|   TEXAS INSTRUMENTS INCORPORATED
|   Standard Linear and Logic
|   IBIS Model of SN74LVTH16244A
|   3.3-V ABT 16-BIT BUFFERS/DRIVERS
|   WITH 3-STATE OUTPUTS
|   TSSOP 48-pin package (DGG)
|   TVSOP 48-pin package (DGV)
|   SSOP 48-pin package (DL)
|   VFBGA 56-pin package (GQL)
[IBIS Ver]   3.2
[Comment char] |_char
[File Name]   sn74lvth16244a.ibs
[File Rev]   1.2 | a_die
[Date]   12/08/04
[Source]   File originated at Texas Instruments, Inc
[Notes]   The following is a sample IBIS file for the SN74LVTH16244A.
   - FILE REV HISTORY
   - 1.2 Re-Release IBIS file on 12/30/04
|   - All test data contained in this file are derived from
|   actual measurement.
|   - The measurement used DGG package.
|   - We have data across voltage and temperature, but not across
|   process.
|   - Since this is a BiCMOS process, we have irregular trend for the
|   curves at high and low temperatures. This data was taken with
|   high temperature for strong case and low for weak case.
|   - Due to presence of BUS-HOLD at input, GND-CLAMP curves
|   have non-monotonic warnings.
|   - Due to the fact that the Device is 5-V Input/Output
|   tolarent, the output model has some Non-Monotonic Warnings.
|   - Power clamp data deleted as there is no power-clamp diode.
|   - File created by Nobuhisa Ohtsubo, TIJ SLL Product Engineering.
|*   Property of Texas Instruments Incorporated.  Unauthorized   *
|*   reproduction and/or distribution is strictly prohibited.   *
|*   This product is protected under copyright law.   *
|*   Created 1998, (C) Copyright 1998, Texas Instruments Inc.,   *
|*   All Rights Reserved   *
|*   UNLESS THERE IS A SIGNED, WRITTEN AGREEMENT TO THE   *
|*   CONTRARY, TEXAS INSTRUMENTS ("TI") IS PROVIDING THE SPICE   *
|*   MODELS "AS IS" AND WITHOUT ANY WARRANTY, EXPRESSED OR   *
|*   IMPLIED.  TI assumes no liability for:   *
|*   1) the accuracy of the IBIS models provided to your   *
|*   company;   *
|*   2) the proper functioning of these IBIS models in your   *
|*   design or for any resulting applications; or   *
|*   3) infringement of patents, copyrights or intellectual   *
|*   property rights resulting from your use of these   *
|*   IBIS models.   *
|*   TI provides IBIS Models as a service to our customers.   *
|*   You and your company shall not distribute, sell or give   *
|*   these models to anyone else without prior written   *
|*   permission from TI.   *
|*   TI reserves the right to make changes to our products or   *
|*   to discontinue any semiconductor product or service   *
|*   without notice, and advises our customers to obtain the   *
|*   latest version of relevant information to verify, before   *
|*   placing orders, that the information being relied on is   *
|*   current.   *
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[Component]   LVTH16244A_DGG
[manufacturer]   Texas Instruments, Inc.
[Package]
|   typ   min   max
R_pkg   0.044   0.038   0.051
L_pkg   3.019nH   2.486nH   4.099nH
C_pkg   0.507pF   0.334pF   0.809pF
[Pin] signal_name  model_name   R_pin   L_pin   C_pin
1   1NOE   LVTH16244A_OE   0.041   4.017nH   0.759pF
2   1Y1   LVTH16244A_OUT   0.042   3.737nH   0.792pF
3   1Y2   LVTH16244A_OUT   0.042   3.48nH   0.661pF
4   GND   GND   0.038   3.131nH   0.575pF
5   1Y3   LVTH16244A_OUT   0.047   3.122nH   0.566pF
6   1Y4   LVTH16244A_OUT   0.043   2.948nH   0.504pF
7   VCC   POWER   0.045   2.845nH   0.397pF
8   2Y1   LVTH16244A_OUT   0.049   2.835nH   0.394pF
9   2Y2   LVTH16244A_OUT   0.048   2.715nH   0.378pF
10   GND   GND   0.050   2.664nH   0.363pF
11   2Y3   LVTH16244A_OUT   0.050   2.585nH   0.348pF
12   2Y4   LVTH16244A_OUT   0.049   2.55nH   0.337pF
13   3Y1   LVTH16244A_OUT   0.049   2.541nH   0.336pF
14   3Y2   LVTH16244A_OUT   0.050   2.574nH   0.348pF
15   GND   GND   0.049   2.618nH   0.359pF
16   3Y3   LVTH16244A_OUT   0.046   2.671nH   0.375pF
17   3Y4   LVTH16244A_OUT   0.045   2.754nH   0.389pF
18   VCC   POWER   0.044   2.823nH   0.450pF
19   4Y1   LVTH16244A_OUT   0.042   2.968nH   0.503pF
20   4Y2   LVTH16244A_OUT   0.051   3.108nH   0.535pF
21   GND   GND   0.042   3.175nH   0.587pF
22   4Y3   LVTH16244A_OUT   0.041   3.449nH   0.678pF
23   4Y4   LVTH16244A_OUT   0.044   3.766nH   0.804pF
24   4NOE   LVTH16244A_OE   0.043   4.065nH   0.761pF
25   3NOE   LVTH16244A_OE   0.041   3.994nH   0.757pF
26   4A4   LVTH16244A_IN   0.039   3.649nH   0.789pF
27   4A3   LVTH16244A_IN   0.038   3.362nH   0.660pF
28   GND   GND   0.038   3.082nH   0.574pF
29   4A2   LVTH16244A_IN   0.044   2.99nH   0.522pF
30   4A1   LVTH16244A_IN   0.041   2.917nH   0.495pF
31   VCC   POWER   0.043   2.82nH   0.448pF
32   3A4   LVTH16244A_IN   0.043   2.699nH   0.385pF
33   3A3   LVTH16244A_IN   0.045   2.628nH   0.372pF
34   GND   GND   0.046   2.556nH   0.356pF
35   3A2   LVTH16244A_IN   0.046   2.495nH   0.344pF
36   3A1   LVTH16244A_IN   0.047   2.487nH   0.334pF
37   2A4   LVTH16244A_IN   0.047   2.49nH   0.335pF
38   2A3   LVTH16244A_IN   0.046   2.486nH   0.343pF
39   GND   GND   0.045   2.566nH   0.356pF
40   2A2   LVTH16244A_IN   0.044   2.639nH   0.374pF
41   2A1   LVTH16244A_IN   0.043   2.701nH   0.386pF
42   VCC   POWER   0.043   2.817nH   0.450pF
43   1A4   LVTH16244A_IN   0.041   2.935nH   0.501pF
44   1A3   LVTH16244A_IN   0.047   3.035nH   0.529pF
45   GND   GND   0.043   3.171nH   0.589pF
46   1A2   LVTH16244A_IN   0.040   3.415nH   0.682pF
47   1A1   LVTH16244A_IN   0.043   3.741nH   0.809pF
48   2NOE   LVTH16244A_OE   0.044   4.099nH   0.764pF
|   TVSOP  48-pin (DGV) package
[Component]   LVTH16244A_DGV
[manufacturer]   Texas   Instruments, Inc.
[Package]
|   typ   min   max
R_pkg   0.063   0.043   0.09
L_pkg   3.077nH   2.377nH   4.305nH
C_pkg   0.387pF   0.281pF   0.565pF
[Pin] signal_name   model_name   R_pin   L_pin   C_pin
1   1NOE   LVTH16244A_OE   0.082   4.277nH   0.562pF
2   1Y1   LVTH16244A_OUT   0.090   4.02nH   0.554pF
3   1Y2   LVTH16244A_OUT   0.087   3.719nH   0.478pF
4   GND   GND   0.087   3.456nH   0.417pF
5   1Y3   LVTH16244A_OUT   0.076   3.207nH   0.411pF
6   1Y4   LVTH16244A_OUT   0.044   2.929nH   0.390pF
7   VCC   POWER   0.046   2.803nH   0.335pF
8   2Y1   LVTH16244A_OUT   0.047   2.683nH   0.321pF
9   2Y2   LVTH16244A_OUT   0.048   2.579nH   0.311pF
10   GND   GND   0.049   2.505nH   0.302pF
11   2Y3   LVTH16244A_OUT   0.048   2.4nH   0.289pF
12   2Y4   LVTH16244A_OUT   0.051   2.4nH   0.283pF
13   3Y1   LVTH16244A_OUT   0.051   2.4nH   0.283pF
14   3Y2   LVTH16244A_OUT   0.050   2.433nH   0.291pF
15   GND   GND   0.048   2.46nH   0.298pF
16   3Y3   LVTH16244A_OUT   0.048   2.585nH   0.312pF
17   3Y4   LVTH16244A_OUT   0.046   2.652nH   0.319pF
18   VCC   POWER   0.045   2.787nH   0.336pF
19   4Y1   LVTH16244A_OUT   0.046   2.962nH   0.394pF
20   4Y2   LVTH16244A_OUT   0.074   3.208nH   0.409pF
21   GND   GND   0.087   3.488nH   0.417pF
22   4Y3   LVTH16244A_OUT   0.087   3.741nH   0.478pF
23   4Y4   LVTH16244A_OUT   0.089   3.99nH   0.546pF
24   4NOE   LVTH16244A_OE   0.084   4.305nH   0.557pF
25   3NOE   LVTH16244A_OE   0.082   4.286nH   0.565pF
26   4A4   LVTH16244A_IN   0.086   3.933nH   0.554pF
27   4A3   LVTH16244A_IN   0.086   3.699nH   0.475pF
28   GND   GND   0.089   3.522nH   0.420pF
29   4A2   LVTH16244A_IN   0.079   3.234nH   0.413pF
30   4A1   LVTH16244A_IN   0.043   2.88nH   0.385pF
31   VCC   POWER   0.045   2.779nH   0.332pF
32   3A4   LVTH16244A_IN   0.045   2.636nH   0.317pF
33   3A3   LVTH16244A_IN   0.047   2.553nH   0.309pF
34   GND   GND   0.048   2.468nH   0.298pF
35   3A2   LVTH16244A_IN   0.050   2.424nH   0.290pF
36   3A1   LVTH16244A_IN   0.050   2.377nH   0.281pF
37   2A4   LVTH16244A_IN   0.050   2.387nH   0.281pF
38   2A3   LVTH16244A_IN   0.050   2.431nH   0.290pF
39   GND   GND   0.048   2.475nH   0.299pF
40   2A2   LVTH16244A_IN   0.048   2.557nH   0.309pF
41   2A1   LVTH16244A_IN   0.047   2.671nH   0.319pF
42   VCC   POWER   0.046   2.804nH   0.334pF
43   1A4   LVTH16244A_IN   0.044   2.935nH   0.390pF
44   1A3   LVTH16244A_IN   0.074   3.203nH   0.412pF
45   GND   GND   0.085   3.444nH   0.416pF
46   1A2   LVTH16244A_IN   0.085   3.723nH   0.477pF
47   1A1   LVTH16244A_IN   0.090   4.012nH   0.547pF
48   2NOE   LVTH16244A_OE   0.083   4.288nH   0.558pF
|   SSOP 48-pin (DL) package
[Component]   LVTH16244A_DL
[manufacturer]   Texas Instruments, Inc.
[Package]
|   typ   min   max
R_pkg   0.048   0.038   0.053
L_pkg   6.046nH   5.084nH   7.968nH
C_pkg   0.813pF   0.569pF   1.157pF
[Pin] signal_name   model_name   R_pin   L_pin   C_pin
1   1NOE   LVTH16244A_OE   0.046   7.968nH   1.017pF
2   1Y1   LVTH16244A_OUT   0.044   7.299nH   1.157pF
3   1Y2   LVTH16244A_OUT   0.043   6.765nH   1.058pF
4   GND   GND   0.041   6.269nH   0.933pF
5   1Y3   LVTH16244A_OUT   0.038   5.856nH   0.829pF
6   1Y4   LVTH16244A_OUT   0.046   5.802nH   0.790pF
7   VCC   POWER   0.050   5.656nH   0.738pF
8   2Y1   LVTH16244A_OUT   0.053   5.5nH   0.643pF
9   2Y2   LVTH16244A_OUT   0.052   5.304nH   0.606pF
10   GND   GND   0.053   5.189nH   0.583pF
11   2Y3   LVTH16244A_OUT   0.051   5.084nH   0.569pF
12   2Y4   LVTH16244A_OUT   0.053   5.862nH   0.833pF
13   3Y1   LVTH16244A_OUT   0.053   5.862nH   0.833pF
14   3Y2   LVTH16244A_OUT   0.051   5.084nH   0.569pF
15   GND   GND   0.053   5.189nH   0.583pF
16   3Y3   LVTH16244A_OUT   0.052   5.304nH   0.606pF
17   3Y4   LVTH16244A_OUT   0.053   5.5nH   0.643pF
18   VCC   POWER   0.050   5.656nH   0.738pF
19   4Y1   LVTH16244A_OUT   0.046   5.802nH   0.790pF
20   4Y2   LVTH16244A_OUT   0.038   5.856nH   0.829pF
21   GND   GND   0.041   6.269nH   0.933pF
22   4Y3   LVTH16244A_OUT   0.043   6.765nH   1.058pF
23   4Y4   LVTH16244A_OUT   0.044   7.299nH   1.157pF
24   4NOE   LVTH16244A_OE   0.046   7.968nH   1.017pF
25   3NOE   LVTH16244A_OE   0.046   7.968nH   1.017pF
26   4A4   LVTH16244A_IN   0.044   7.299nH   1.157pF
27   4A3   LVTH16244A_IN   0.043   6.765nH   1.058pF
28   GND   GND   0.041   6.269nH   0.933pF
29   4A2   LVTH16244A_IN   0.038   5.856nH   0.829pF
30   4A1   LVTH16244A_IN   0.046   5.802nH   0.790pF
31   VCC   POWER   0.050   5.656nH   0.738pF
32   3A4   LVTH16244A_IN   0.053   5.5nH   0.643pF
33   3A3   LVTH16244A_IN   0.052   5.304nH   0.606pF
34   GND   GND   0.053   5.189nH   0.583pF
35   3A2   LVTH16244A_IN   0.051   5.084nH   0.569pF
36   3A1   LVTH16244A_IN   0.053   5.862nH   0.833pF
37   2A4   LVTH16244A_IN   0.053   5.862nH   0.833pF
38   2A3   LVTH16244A_IN   0.051   5.084nH   0.569pF
39   GND   GND   0.053   5.189nH   0.583pF
40   2A2   LVTH16244A_IN   0.052   5.304nH   0.606pF
41   2A1   LVTH16244A_IN   0.053   5.5nH   0.643pF
42   VCC   POWER   0.005   5.656nH   0.738pF
43   1A4   LVTH16244A_IN   0.046   5.802nH   0.790pF
44   1A3   LVTH16244A_IN   0.038   5.856nH   0.829pF
45   GND   GND   0.041   6.269nH   0.933pF
46   1A2   LVTH16244A_IN   0.043   6.765nH   1.058pF
47   1A1   LVTH16244A_IN   0.044   7.299nH   1.157pF
48   2NOE   LVTH16244A_OE   0.046   7.967nH   1.017pF
| Component LVTH16244A_GQL 48-pin VFBGA
[Component]   LVTH16244A_GQL
[Manufacturer]   Texas Instruments, Inc.
[Package]
|   typ   min   max
R_pkg   7.900e-02   4.500e-02   9.400e-02
L_pkg   2.264e-09   1.398e-09   2.722e-09
C_pkg   3.060e-13   1.170e-13   4.040e-13
[Pin]   signal_name   model_name   R_pin   L_pin   C_pin
A1   1NOE   LVTH16244A_OE   5.100e-02   1.531e-09   2.100e-13
B2   1Y1   LVTH16244A_OUT   7.300e-02   2.572e-09   3.120e-13
B1   1Y2   LVTH16244A_OUT   7.100e-02   1.835e-09   2.320e-13
B3   GND   GND   9.400e-02   2.717e-09   3.830e-13
C2   1Y3   LVTH16244A_OUT   8.900e-02   2.534e-09   3.500e-13
C1   1Y4   LVTH16244A_OUT   7.100e-02   1.831e-09   2.310e-13
C3   VCC   POWER   9.400e-02   2.722e-09   3.920e-13
D2   2Y1   LVTH16244A_OUT   9.000e-02   2.551e-09   3.520e-13
D1   2Y2   LVTH16244A_OUT   7.200e-02   1.846e-09   2.440e-13
D3   GND   GND   9.400e-02   2.719e-09   4.030e-13
E2   2Y3   LVTH16244A_OUT   8.900e-02   2.541e-09   3.510e-13
E1   2Y4   LVTH16244A_OUT   7.200e-02   1.850e-09   2.270e-13
F1   3Y1   LVTH16244A_OUT   7.200e-02   1.850e-09   2.270e-13
F2   3Y2   LVTH16244A_OUT   8.900e-02   2.541e-09   3.510e-13
G3   GND   GND   9.400e-02   2.718e-09   4.040e-13
G1   3Y3   LVTH16244A_OUT   7.200e-02   1.847e-09   2.440e-13
G2   3Y4   LVTH16244A_OUT   9.000e-02   2.551e-09   3.520e-13
H3   VCC   POWER   9.400e-02   2.721e-09   3.920e-13
H1   4Y1   LVTH16244A_OUT   7.000e-02   1.830e-09   2.310e-13
H2   4Y2   LVTH16244A_OUT   8.800e-02   2.524e-09   3.500e-13
J3   GND   GND   9.300e-02   2.709e-09   3.820e-13
J1   4Y3   LVTH16244A_OUT   7.100e-02   1.851e-09   2.330e-13
J2   4Y4   LVTH16244A_OUT   5.600e-02   2.605e-09   3.900e-13
K1   4NOE   LVTH16244A_OE   4.500e-02   1.398e-09   1.170e-13
K6   3NOE   LVTH16244A_OE   4.500e-02   1.512e-09   1.930e-13
J5   4A4   LVTH16244A_IN   5.500e-02   2.492e-09   3.130e-13
J6   4A3   LVTH16244A_IN   7.000e-02   1.821e-09   2.300e-13
J4   GND   GND   9.300e-02   2.703e-09   3.820e-13
H5   4A2   LVTH16244A_IN   8.900e-02   2.529e-09   3.500e-13
H6   4A1   LVTH16244A_IN   7.100e-02   1.826e-09   2.300e-13
H4   VCC   POWER   9.400e-02   2.722e-09   3.910e-13
G5   3A4   LVTH16244A_IN   9.000e-02   2.551e-09   3.520e-13
G6   3A3   LVTH16244A_IN   7.200e-02   1.846e-09   2.440e-13
G4   GND   GND   9.400e-02   2.719e-09   4.040e-13
F5   3A2   LVTH16244A_IN   8.800e-02   2.510e-09   3.490e-13
F6   3A1   LVTH16244A_IN   7.200e-02   1.850e-09   2.270e-13
E6   2A4   LVTH16244A_IN   7.100e-02   1.850e-09   2.270e-13
E5   2A3   LVTH16244A_IN   8.900e-02   2.529e-09   3.500e-13
D4   GND   GND   9.400e-02   2.719e-09   4.030e-13
D6   2A2   LVTH16244A_IN   7.200e-02   1.847e-09   2.430e-13
D5   2A1   LVTH16244A_IN   8.900e-02   2.550e-09   3.520e-13
C4   VCC   POWER   9.400e-02   2.722e-09   3.910e-13
C6   1A4   LVTH16244A_IN   7.100e-02   1.827e-09   2.300e-13
C5   1A3   LVTH16244A_IN   8.900e-02   2.539e-09   3.500e-13
B4   GND   GND   9.300e-02   2.705e-09   3.820e-13
B6   1A2   LVTH16244A_IN   7.100e-02   1.831e-09   2.270e-13
B5   1A1   LVTH16244A_IN   7.300e-02   2.685e-09   3.800e-13
A6   2NOE   LVTH16244A_OE   5.100e-02   1.417e-09   1.330e-13
[Model Selector]   LVTH16244A_IN
LVTH16244A_IN_28   2.8-V Vcc Input Model
LVTH16244A_IN_33   3.3-V Vcc Input Model
[Model Selector]   LVTH16244A_OE
LVTH16244A_OE_28   2.8-V Vcc Input Model
LVTH16244A_OE_33   3.3-V Vcc Input Model
[Model Selector]   LVTH16244A_OUT
LVTH16244A_OUT_28   2.8-V Vcc Output Model
LVTH16244A_OUT_33   3.3-V Vcc Output Model
| Models and submodels in the file (6): LVTH16244A_OUT_28 (3-state), LVTH16244A_OE_28 (Input), LVTH16244A_IN_28 (Input), LVTH16244A_OUT_33 (3-state), LVTH16244A_OE_33 (Input), LVTH16244A_IN_33 (Input)
